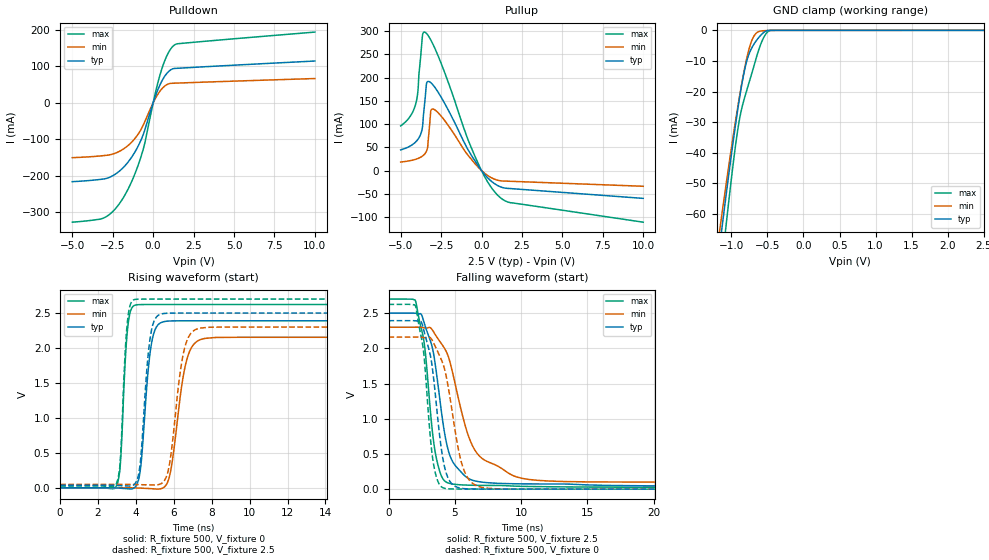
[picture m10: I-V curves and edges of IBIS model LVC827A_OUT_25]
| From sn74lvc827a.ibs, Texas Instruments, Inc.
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[Model]   LVC827A_OUT_25
Model_type  3-state
Enable   Active-Low
Vref =   0
Rref =   500
Cref =   30p
Vmeas =   1.25
| variable   typ   min   max
C_comp   5.92pF   5.29pF   6.91pF
| C_pullup   7.37pF   6.40pF   7.97pF
| C_pulldown   10.26pF   6.97pF   15.74pF
| C_tri-state   5.92pF   5.29pF   6.91pF
[Temperature Range]   40   100   -40
| Ambient temperature   25   85   -40
[Voltage range]   2.5   2.3   2.7
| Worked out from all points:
|   slope of the pulldown table from 0 to 0.375 V, typ, clamps not added: 8.36 ohm
|   slope of the pullup table from 0 to 0.375 V, typ, clamps not added: 24.4 ohm
|   GND clamp passes 1 mA (typ) near -0.57 V on its own axis
|   rising waveform, R_fixture 500, V_fixture 0: 20-80 % time 423ps typ, 642ps min, 283ps max; typ from 0 V to 2.39 V
|   falling waveform, R_fixture 500, V_fixture 2.5: 20-80 % time 1.23ns typ, 2.15ns min, 881ps max; typ from 2.5 V to 0.036 V
|   rising waveform, R_fixture 500, V_fixture 2.5: 20-80 % time 401ps typ, 594ps min, 274ps max; typ from 0.036 V to 2.5 V
|   falling waveform, R_fixture 500, V_fixture 0: 20-80 % time 925ps typ, 1.23ns min, 742ps max; typ from 2.39 V to 0 V
[GND Clamp]
| LVC827A_OUT_25
|   Voltage   I(typ)   I(min)   I(max)
-5V       -931.5mA   -844.2mA   -1.078A
-1.17V    -72.22mA   -66.78mA   -84.97mA
-1.135V   -65.53mA   -60.79mA   -77.21mA
-1.07V    -53.37mA   -49.89mA   -63.11mA
-915mV    -26.52mA   -25.66mA   -33.14mA
-860mV    -18.37mA   -18mA      -25.97mA
-795mV    -10.82mA   -10.09mA   -20.28mA
-735mV    -6.635mA   -4.578mA   -15.56mA
-670mV    -3.933mA   -1.323mA   -10.3mA
-580mV    -1.311mA   -195.7uA   -3.823mA
-495mV    -38.55uA   -71.29uA   -493.2uA
2.5V      64.36pA    31.71nA    -986.8pA
[Pulldown]
| LVC827A_OUT_25
|   Voltage   I(typ)   I(min)   I(max)
-5V       -216.2mA   -150.4mA   -327.5mA
-2.98V    -208.2mA   -144.3mA   -314.3mA
-2.365V   -196.4mA   -138.4mA   -292.1mA
-1.755V   -173.1mA   -124mA     -253.6mA
-1.17V    -138mA     -99.98mA   -199.5mA
-645mV    -90.59mA   -63.98mA   -132.2mA
-490mV    -70.77mA   -48.75mA   -105mA
150mV     19.67mA    13.16mA    30.02mA
550mV     60.93mA    39.25mA    95.08mA
920mV     84.62mA    51.74mA    135.9mA
1.29V     94.42mA    54.12mA    158.1mA
10V       115mA      66.94mA    194.5mA
[Pullup]
| LVC827A_OUT_25
|   Voltage   I(typ)   I(min)   I(max)
-5V       44.47mA    18.44mA    96.09mA
-4.06V    61.99mA    24.45mA    144.5mA
-3.935V   67.07mA    25.99mA    170.1mA
-3.685V   87mA       30.45mA    277mA
-3.63V    100mA      31.84mA    293.9mA
-3.5V     150.3mA    36.29mA    297.4mA
-3.375V   189.7mA    44.35mA    293.7mA
-3.14V    189mA      127.8mA    280.9mA
-2.965V   182.5mA    132mA      268.8mA
-390mV    20.16mA    14.42mA    29.44mA
1.125V    -34.24mA   -21.6mA    -56.95mA
10V       -59.7mA    -33.65mA   -110.8mA
[Ramp]
| LVC827A_OUT_25
| variable   typ   min   max
dV/dt_r   1.44/4.32E-10   1.30/6.49E-10   1.58/2.97E-10
dV/dt_f   1.48/1.23E-09   1.35/2.15E-09   1.60/8.85E-10
R_load = 500
[Rising Waveform]
| LVC827A_OUT_25
R_fixture =   500
C_fixture =   0
L_fixture =   0
V_fixture =   0
V_fixture_min = 0
V_fixture_max = 0
|   Time   V(typ)   V(min)   V(max)
0s        497.9pV    2.301nV    14.6nV
2.985ns   -1.476mV   745.5uV    37.83mV
3.18ns    -5.014mV   744.2uV    357.6mV
3.57ns    -13.23mV   714.4uV    2.306V
4.005ns   27.62mV    -1.605mV   2.617V
4.815ns   2.058V     -12.12mV   2.622V
5.5ns     2.378V     12.32mV    2.623V
6.68ns    2.389V     1.832V     2.623V
7.63ns    2.39V      2.137V     2.623V
50ns      2.39V      2.154V     2.623V
[Falling Waveform]
| LVC827A_OUT_25
R_fixture =   500
C_fixture =   0
L_fixture =   0
V_fixture =   2.5
V_fixture_min = 2.3
V_fixture_max = 2.7
|   Time   V(typ)   V(min)   V(max)
0s        2.5V       2.3V       2.7V
2.04ns    2.498V     2.3V       2.671V
2.71ns    2.35V      2.291V     2.05V
3.56ns    1.728V     2.186V     489.2mV
4.165ns   872.9mV    2.018V     131.6mV
4.585ns   503.8mV    1.84V      82.92mV
5.77ns    186.9mV    913.9mV    58.77mV
6.51ns    117.9mV    556.6mV    54.93mV
10.07ns   75.61mV    154mV      40.03mV
50ns      36.06mV    50.67mV    25.63mV
[Rising Waveform]
| LVC827A_OUT_25
R_fixture =   500
C_fixture =   0
L_fixture =   0
V_fixture =   2.5
V_fixture_min = 2.3
V_fixture_max = 2.7
|   Time   V(typ)   V(min)   V(max)
0s        35.95mV    48.94mV    25.63mV
2.98ns    34.43mV    49.52mV    68.55mV
3.17ns    31.47mV    49.45mV    384.3mV
3.535ns   26.8mV     49.33mV    2.338V
3.925ns   52.04mV    47.74mV    2.694V
4.775ns   2.188V     42.36mV    2.7V
5.395ns   2.49V      71.67mV    2.7V
6.555ns   2.5V       1.986V     2.7V
7.405ns   2.5V       2.286V     2.7V
50ns      2.5V       2.3V       2.7V
[Falling Waveform]
| LVC827A_OUT_25
R_fixture =   500
C_fixture =   0
L_fixture =   0
V_fixture =   0
V_fixture_min = 0
V_fixture_max = 0
|   Time   V(typ)   V(min)   V(max)
0s        2.393V     2.159V     2.625V
2.045ns   2.391V     2.159V     2.596V
2.65ns    2.267V     2.153V     1.943V
3.13ns    1.921V     2.155V     787.4mV
3.375ns   1.62V      2.087V     382.3mV
4.205ns   335.9mV    1.722V     13.19mV
4.695ns   94.55mV    1.234V     3.822mV
5.58ns    9.82mV     331.1mV    1.655mV
7.09ns    1.827mV    23.62mV    667.9uV
50ns      20.71uV    122.1uV    5.402uV
